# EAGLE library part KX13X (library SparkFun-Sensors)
Kionix KX134 Tri-Axis Accelerometer The KX134-1211 is a tri-axis ±8g, ±16g, ±32g, or ±64g silicon micromachined accelerometer featuring a user-configurable 3-stage Advanced Data Path (ADP) consisting of a low-pass filter, low-pass/high-pass filter, and RMS calculation engine. The KX134-1211 accelerometer also features an advanced Wake-Up and Back-to-Sleep detection with a high-resolution threshold capability configurable down to 15.6 mg, 512-byte buffer that continues to record data even when being read, as well as embedded engines for orientation, Directional-TapTM/DoubleTapTM, and Free fall detection.
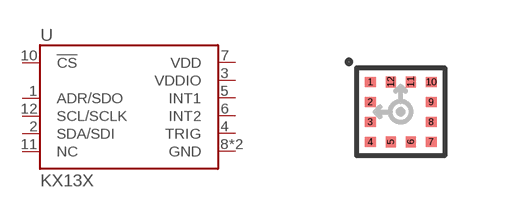
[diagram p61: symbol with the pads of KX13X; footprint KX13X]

Designator prefix U

## KX13X-KX134 (PROD_ID: IC-15486; VALUE: KX134)  [KX13X]
1  ADR/SDO
2  SDA/SDI
3  VDDIO
4  TRIG
5  INT1
6  INT2
7  VDD
8  GND
9  GND
10  !CS
11  NC  nc
12  SCL/SCLK

## KX13X-KX132 (PROD_ID: IC-15721; VALUE: KX132)  [KX13X]
Pads as for KX13X

## Footprint KX13X (pad centres in mm)
Kionix KX134 Tri-Axis Accelerometer The KX134-1211 is a tri-axis ±8g, ±16g, ±32g, or ±64g silicon micromachined accelerometer featuring a user-configurable 3-stage Advanced Data Path (ADP) consisting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
smd 0.275 x 0.25: 1 -0.762,0.75; 2 -0.762,0.25; 3 -0.762,-0.25; 4 -0.762,-0.75; 7 0.762,-0.75; 8 0.762,-0.25; 9 0.762,0.25; 10 0.762,0.75
smd 0.25 x 0.275: 5 -0.25,-0.75; 6 0.25,-0.75; 11 0.25,0.75; 12 -0.25,0.75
